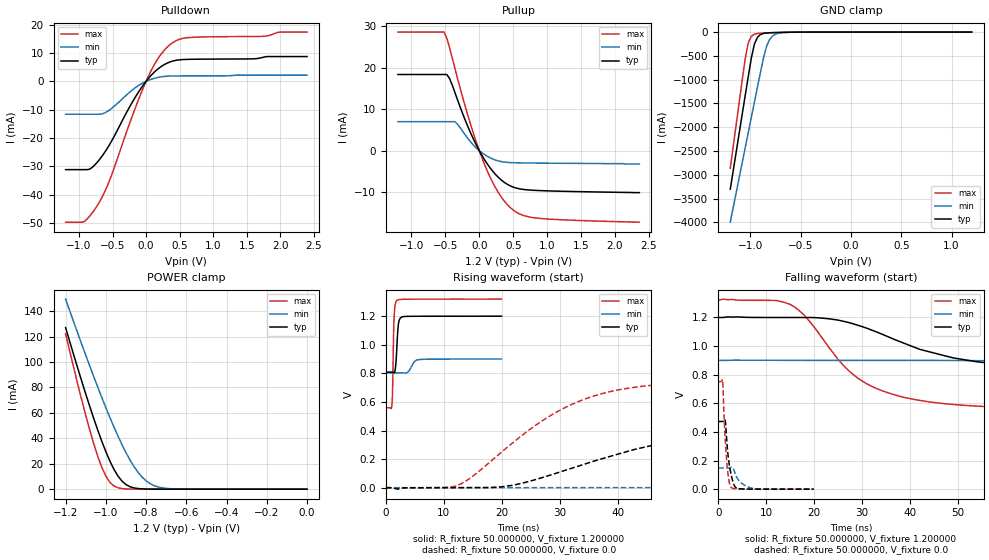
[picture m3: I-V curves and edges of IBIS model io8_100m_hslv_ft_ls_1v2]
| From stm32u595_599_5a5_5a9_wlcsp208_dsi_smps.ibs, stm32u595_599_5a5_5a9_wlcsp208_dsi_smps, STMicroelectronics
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|   Model io8_100m_hslv_ft_ls_1v2
[Model]  io8_100m_hslv_ft_ls_1v2
Model_type I/O
Polarity   Non-Inverting
Enable   Active-Low
Vinl =   0.360000V
Vinh =   0.840000V
Vmeas =  0.600000V
Cref =   50.000000pF
Rref =   100.000000M
Vref =   0.0V
C_comp   3.030000pF   2.960800pF   3.078200pF
[Temperature Range]   25.000000   0.140000k   -40.000000
[Pullup Reference]   1.200000V   0.900000V   1.320000V
[Pulldown Reference]   0.0V   0.0V   0.0V
[POWER Clamp Reference]   1.200000V   0.900000V   1.320000V
[GND Clamp Reference]   0.0V   0.0V   0.0V
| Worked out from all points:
|   slope of the pulldown table from 0 to 0.18 V, typ, clamps not added: 40.7 ohm
|   slope of the pullup table from 0 to 0.18 V, typ, clamps not added: 39.5 ohm
|   GND clamp passes 1 mA (typ) near -0.51 V on its own axis
|   POWER clamp passes 1 mA (typ) near -0.86 V on its own axis
|   rising waveform, R_fixture 50.000000, V_fixture 1.200000: 20-80 % time 346ps typ, 819ps min, 226ps max; typ from 0.809 V to 1.2 V
|   rising waveform, R_fixture 50.000000, V_fixture 0.0: 20-80 % time 27.9ns typ, 68.2ns min, 16ns max; typ from 0 V to 0.473 V
|   falling waveform, R_fixture 50.000000, V_fixture 1.200000: 20-80 % time 23.6ns typ, 56.9ns min, 13.3ns max; typ from 1.2 V to 0.809 V
|   falling waveform, R_fixture 50.000000, V_fixture 0.0: 20-80 % time 1.04ns typ, 1.96ns min, 792ps max; typ from 0.473 V to 0 V
[Pulldown]
|Voltage   I(typ)   I(min)   I(max)
-1.2V     -31.16mA   -11.61mA   -49.71mA
-920mV    -31.16mA   -11.61mA   -49.48mA
-840mV    -31mA      -11.61mA   -47.54mA
-720mV    -28.32mA   -11.61mA   -43.58mA
-560mV    -22.95mA   -10.36mA   -35.89mA
-200mV    -7.146mA   -2.962mA   -11.89mA
0V        0A         -1.6pA     0A
160mV     4.047mA    1.297mA    7.361mA
360mV     6.87mA     1.868mA    13mA
640mV     7.764mA    1.921mA    15.46mA
1.76V     8.564mA    2.185mA    15.9mA
2.4V      8.742mA    2.185mA    17.38mA
[Pullup]
|Voltage   I(typ)   I(min)   I(max)
-1.2V     18.39mA    7.011mA    28.62mA
-520mV    18.39mA    7.011mA    28.62mA
-440mV    17.47mA    7.011mA    24.94mA
-360mV    14.06mA    7.011mA    19.88mA
-160mV    5.494mA    2.765mA    8.045mA
40mV      -1.16mA    -507.9uA   -1.774mA
240mV     -5.73mA    -2.255mA   -8.953mA
360mV     -7.518mA   -2.714mA   -11.96mA
480mV     -8.639mA   -2.875mA   -14.04mA
640mV     -9.31mA    -2.939mA   -15.55mA
880mV     -9.601mA   -2.983mA   -16.29mA
2.36V     -10.1mA    -3.2mA     -17.23mA
[GND_clamp]
|Voltage   I(typ)   I(min)   I(max)
-1.2V     -3.305A    -3.998A    -2.862A
-1.05V    -1.316A    -2.418A    -539.3mA
-1.02V    -921mA     -2.103A    -218.8mA
-990mV    -539.5mA   -1.788A    -87.43mA
-960mV    -252.1mA   -1.474A    -44.36mA
-930mV    -110.5mA   -1.16A     -30.32mA
-870mV    -28.03mA   -549.1mA   -21.09mA
-840mV    -18.43mA   -305.6mA   -18.27mA
-810mV    -13.9mA    -159.7mA   -15.73mA
-780mV    -11.23mA   -82.35mA   -13.37mA
-600mV    -2.976mA   -4.272mA   -3.058mA
1.2V      0A         14.73nA    0A
[POWER_clamp]
|Voltage   I(typ)   I(min)   I(max)
-1.2V     127mA      149.4mA    122.2mA
-1.12V    84.97mA    114mA      70.27mA
-1.06V    55.51mA    88.42mA    35.67mA
-1.02V    37.63mA    72.04mA    17.17mA
-1V       29.51mA    64.13mA    10.3mA
-960mV    15.69mA    48.99mA    2.571mA
-900mV    3.624mA    28.77mA    182.8uA
-840mV    490.7uA    13.24mA    11.35uA
-800mV    116.8uA    6.532mA    1.77uA
-740mV    13.2uA     1.723mA    109.1nA
-620mV    167.3nA    79.35uA    0A
0V        0A         17.84nA    0A
[Ramp]
| variable   typ   min   max
dV/dt_r  0.28372/27.87645n   88.79987m/68.15740n 0.45094/16.00557n
dV/dt_f  0.23464/23.61960n   57.84000m/56.86431n 0.45665/13.31082n
R_load = 50.000000
[Rising Waveform]
R_fixture= 50.000000
V_fixture= 1.200000
V_fixture_min= 0.900000
V_fixture_max= 1.320000
|time   V(typ)   V(min)   V(max)
0s        809mV      803.6mV    558.9mV
1.041ns   809.1mV    803.6mV    576.2mV
1.161ns   808.6mV    803.6mV    689.4mV
1.321ns   805.8mV    803.6mV    1.049V
1.441ns   803.6mV    803.6mV    1.208V
1.922ns   1.004V     803.6mV    1.311V
2.242ns   1.163V     803.7mV    1.316V
2.843ns   1.196V     803.4mV    1.318V
5.726ns   1.2V       896mV      1.319V
19.94ns   1.2V       900mV      1.32V
[Rising Waveform]
R_fixture= 50.000000
V_fixture= 0.0
V_fixture_min= 0.0
V_fixture_max= 0.0
|time   V(typ)   V(min)   V(max)
0s        2.231nV    213nV      1.42nV
13.01ns   -87.74uV   -84.37uV   27.87mV
20.02ns   6.343mV    -72.45uV   251mV
26.03ns   58.91mV    -40.83uV   442.2mV
35.04ns   174.6mV    97.55uV    630.4mV
44.04ns   278.2mV    305.2uV    708.9mV
56.06ns   373.5mV    2.315mV    740.8mV
90.09ns   461.4mV    43.74mV    751.3mV
193.2ns   472.8mV    139.4mV    751.5mV
498.5ns   472.9mV    148.1mV    751.6mV
[Falling Waveform]
R_fixture= 50.000000
V_fixture= 1.200000
V_fixture_min= 0.900000
V_fixture_max= 1.320000
|time   V(typ)   V(min)   V(max)
0s        1.2V       900mV      1.32V
15.02ns   1.2V       900.2mV    1.292V
18.02ns   1.2V       900.1mV    1.213V
27.03ns   1.167V     900mV      834.3mV
34.03ns   1.085V     900mV      690mV
42.04ns   977.7mV    900mV      620.7mV
56.06ns   883.1mV    897.6mV    577.2mV
96.1ns    817.2mV    850.5mV    559.5mV
171.2ns   809.1mV    811mV      558.9mV
498.5ns   809mV      803.6mV    558.9mV
[Falling Waveform]
R_fixture= 50.000000
V_fixture= 0.0
V_fixture_min= 0.0
V_fixture_max= 0.0
|time   V(typ)   V(min)   V(max)
0s        472.9mV    148.1mV    751.6mV
920.9ps   473.3mV    148.2mV    763.1mV
1.201ns   475mV      148.3mV    524.9mV
1.441ns   484.6mV    148.3mV    362.2mV
1.682ns   392.5mV    148.3mV    237.8mV
2.202ns   196.5mV    148.2mV    67.57mV
2.683ns   104.6mV    152.6mV    13.54mV
3.724ns   9.273mV    93.79mV    1.915mV
6.927ns   176.7uV    7.5mV      296.1uV
19.94ns   2.231nV    213nV      1.42nV
